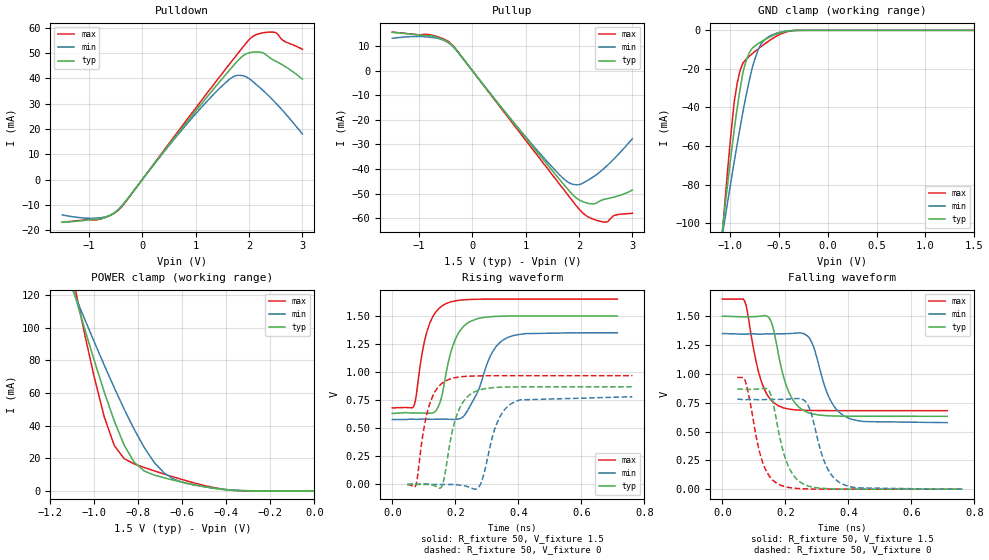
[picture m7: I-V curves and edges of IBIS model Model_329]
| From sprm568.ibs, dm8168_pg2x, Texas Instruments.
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| Model based on original model for BSHTLTCSCDDVGPBFZ
|   Sub model FASTEST_11MA_10PER_P_1P5
[model]   Model_329
|[Description]  [1.5V-3-STATE-X-FASTEST:11MA, IND, 10%]
|   Fastest slew rate (SR[1:0] = "00"), 0.73 * RExt = 1.325 * Iout
|   (I[2:0] = "110"), 11mA nominal with Rext = 50R, ,Industrial
|   temperature range (-40C to 125C, 25C nominal),10% power supply
|   tolerance
|[Input Load]
|[Output Drive] FASTEST:11MA
|Voltage   1.5V
|Mode   3-STATE
Model_type   3-state
Polarity   Non-Inverting
Enable   Active-Low
Cref =  15.0000pF
Rref =  100.0000M
Vref =  0V
Vmeas =  0.75
C_comp   1.5249p   1.4275p   1.6205p
[Model Spec]
[Temperature Range]   25   125   -40
[Voltage Range]   1.5   1.35   1.65
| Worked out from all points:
|   slope of the pulldown table from 0 to 0.225 V, typ, clamps not added: 36.2 ohm
|   slope of the pullup table from 0 to 0.225 V, typ, clamps not added: 36.1 ohm
|   GND clamp passes 1 mA (typ) near -0.47 V on its own axis
|   POWER clamp passes 1 mA (typ) near -0.42 V on its own axis
|   rising waveform, R_fixture 50, V_fixture 1.5: 20-80 % time 47.4ps typ, 68.3ps min, 42.4ps max; typ from 0.633 V to 1.5 V
|   rising waveform, R_fixture 50, V_fixture 0: 20-80 % time 45.1ps typ, 50ps min, 41.3ps max; typ from 0 V to 0.87 V
|   falling waveform, R_fixture 50, V_fixture 1.5: 20-80 % time 50.4ps typ, 57.2ps min, 47.7ps max; typ from 1.5 V to 0.632 V
|   falling waveform, R_fixture 50, V_fixture 0: 20-80 % time 48.9ps typ, 53.2ps min, 46.6ps max; typ from 0.87 V to 0 V
[POWER_clamp]
-1.5V     321.6mA    260.6mA    415.8mA
-1.091V   121.1mA    120.8mA    126.6mA
-1.076V   114.1mA    115.8mA    116.8mA
-1V       79.88mA    91.3mA     69.56mA
-954.5mV  60.58mA    77.05mA    45.34mA
-909.1mV  42.84mA    63.2mA     27.8mA
-818.2mV  17.47mA    37.6mA     16.51mA
-772.7mV  12.19mA    26.53mA    14.33mA
-681.8mV  7.985mA    10.89mA    10.33mA
-590.9mV  5.092mA    4.952mA    6.596mA
-363.6mV  298.9uA    465.6uA    298.1uA
0V        1.518nA    23.05nA    396.5pA
[Pulldown]
-1.5V     -16.86mA   -14.04mA   -16.9mA
-772.7mV  -15.51mA   -15.09mA   -15.55mA
-590.9mV  -14.04mA   -13.99mA   -14.12mA
-409.1mV  -11.11mA   -11mA      -11.35mA
954.5mV   25.91mA    24.89mA    26.98mA
1.455V    38.83mA    36.23mA    40.8mA
1.727V    45.55mA    40.89mA    48.2mA
2V        50.13mA    39.99mA    55.32mA
2.318V    49.42mA    34.17mA    58.25mA
2.5V      46.85mA    30.32mA    58.16mA
2.636V    45.27mA    27.17mA    55.07mA
3V        39.74mA    18.03mA    51.54mA
[Pullup]
-1.5V     15.55mA    13.13mA    15.65mA
-818.2mV  14.19mA    13.62mA    14.67mA
-409.1mV  10.85mA    10.66mA    11.17mA
1.227V    -33.46mA   -32.67mA   -34.7mA
1.682V    -45.43mA   -43.35mA   -47.47mA
1.864V    -50.03mA   -46.07mA   -52.55mA
2V        -52.51mA   -46.33mA   -56.27mA
2.182V    -53.99mA   -44.37mA   -59.58mA
2.409V    -52.78mA   -40.88mA   -61.31mA
2.545V    -51.96mA   -38.24mA   -61.26mA
2.682V    -51.26mA   -35.3mA    -58.71mA
3V        -48.54mA   -27.68mA   -57.97mA
[GND_clamp]
-1.5V     -310mA     -250.5mA   -402.4mA
-1.076V   -103.5mA   -106.1mA   -105.2mA
-1.045V   -89.74mA   -96.32mA   -85.93mA
-954.5mV  -51.19mA   -67.85mA   -36.85mA
-924.2mV  -40.06mA   -58.84mA   -27.27mA
-863.6mV  -21.23mA   -41.55mA   -16.73mA
-833.3mV  -15.79mA   -33.74mA   -15.03mA
-772.7mV  -9.342mA   -19.74mA   -12.19mA
-712.1mV  -6.927mA   -10.35mA   -9.702mA
-621.2mV  -4.26mA    -3.894mA   -6.224mA
-409.1mV  -336.9uA   -288.9uA   -618.6uA
1.5V      1.518nA    2.298uA    269.6pA
[Ramp]
dV/dt_f   0.699024/80.981006p   0.622768/93.510381p   0.777824/74.729977p
dV/dt_r   0.721948/73.493362p  0.6578976/82.534055p  0.7930152/66.439668p
R_load = 50
[Rising Waveform]
R_fixture = 50
V_fixture = 1.5
V_fixture_min = 1.35
V_fixture_max = 1.65
0s        632.9mV    578.1mV    682mV
68.59ps   635.4mV    580.6mV    699.3mV
111.7ps   633.9mV    581.4mV    1.376V
145.4ps   689.3mV    581.1mV    1.558V
169.9ps   976.8mV    581.1mV    1.609V
198.8ps   1.283V     579.1mV    1.633V
232.8ps   1.423V     630.1mV    1.644V
318.1ps   1.494V     1.179V     1.65V
366.9ps   1.499V     1.309V     1.65V
714.3ps   1.5V       1.35V      1.65V
[Rising Waveform]
R_fixture = 50
V_fixture = 0
V_fixture_min = 0
V_fixture_max = 0
47.92ps   0V         0V         0V
74.59ps   0V         2.38mV     -6.849mV
109.4ps   0V         4.15mV     623.4mV
153ps     -31.29mV   0V         888.2mV
179.7ps   314.9mV    0V         935.3mV
214.1ps   680.8mV    -5.482mV   957.2mV
273ps     837.7mV    -29.86mV   966.4mV
337.8ps   864.7mV    581.4mV    968mV
392.9ps   868.4mV    740.6mV    968.3mV
762.2ps   869.6mV    780.8mV    968.5mV
[Falling Waveform]
R_fixture = 50
V_fixture = 1.5
V_fixture_min = 1.35
V_fixture_max = 1.65
0s        1.501V     1.35V      1.649V
70.67ps   1.496V     1.344V     1.634V
123ps     1.502V     1.345V     943.7mV
153.8ps   1.462V     1.347V     777mV
177ps     1.189V     1.348V     724.6mV
212.4ps   834.7mV    1.35V      694.4mV
269.4ps   667.5mV    1.331V     683.5mV
334.6ps   637.1mV    823.2mV    681.6mV
382.4ps   633.4mV    643mV      681.4mV
714.3ps   632.2mV    577.2mV    681.1mV
[Falling Waveform]
R_fixture = 50
V_fixture = 0
V_fixture_min = 0
V_fixture_max = 0
47.92ps   869.9mV    781mV      969.2mV
74.84ps   865.4mV    775.8mV    923.2mV
117.5ps   870.1mV    775.4mV    331.5mV
145.6ps   862.7mV    778.3mV    129.6mV
185.5ps   413.9mV    779.4mV    33.2mV
221.2ps   139.6mV    783.7mV    10.28mV
269.8ps   30.93mV    741mV      2.429mV
328.5ps   5.572mV    210.4mV    0V
380.7ps   0V         44.98mV    0V
762.2ps   0V         0V         0V
